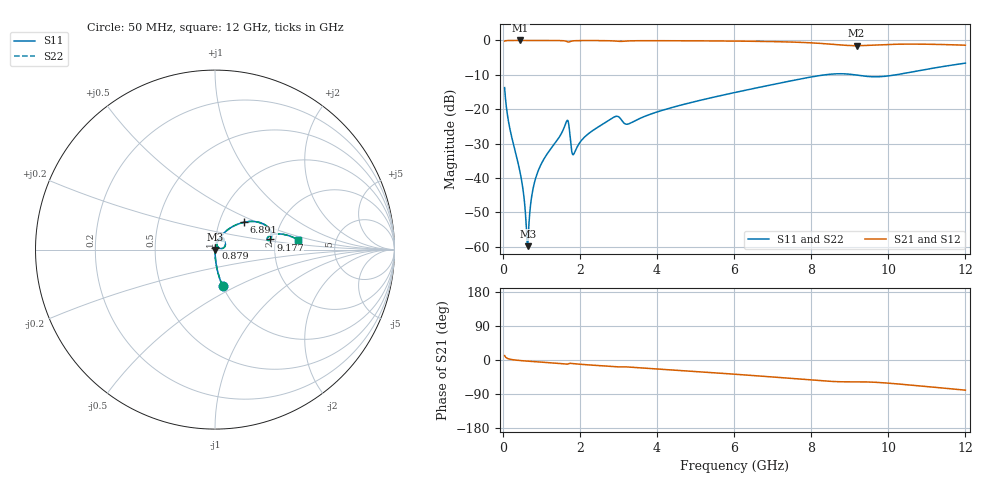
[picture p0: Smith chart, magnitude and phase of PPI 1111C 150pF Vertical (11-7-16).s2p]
# GHz S MA R 50
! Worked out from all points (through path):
!   1601 points, 50 MHz to 12 GHz, reference 50 ohm
!   highest |S21| = -0.01 dB at 453.3 MHz (marker M1); lowest = -1.5 dB at 9.177 GHz (marker M2)
!   group delay of S21, straight-line fit = 18.3 ps
!   lowest |S11| = -59.9 dB at 647.5 MHz (marker M3), VSWR 1.00, Z = 50.1 + j0.0126 ohm
!   |S11| at or under -10 dB: start of sweep to 8.361 GHz; 9.128 GHz to 10.2 GHz (1.071 GHz wide, 11.1 % of centre)
!   |S22| runs from -59.9 to -6.6 dB; largest |S21 - S12| = 0
!   S11 on the Smith chart (normalised r, x): 50 MHz: 1.00, -0.42; 879 MHz: 1.00, +0.02; 6.891 GHz: 1.31, +0.42; 9.177 GHz: 1.87, +0.24; 12 GHz: 2.70, +0.37
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0.05  0.2058 -78.3  0.9782 11.6  0.9782 11.6  0.2058 -78.3
0.1844375  0.05266 -87.2  0.998 2.2  0.998 2.2  0.05266 -87.2
0.4533125  0.01192 -87.4  0.9991 -1.4  0.9991 -1.4  0.01192 -87.4
0.5354688  0.006254 -83.7  0.999 -2.1  0.999 -2.1  0.006254 -83.7
0.6101562  0.002056 -64.5  0.999 -2.7  0.999 -2.7  0.002056 -64.5
0.6475  0.001017 7.1  0.999 -3.0  0.999 -3.0  0.001017 7.1
0.6848437  0.002311 60.2  0.9989 -3.3  0.9989 -3.3  0.002311 60.2
0.7744688  0.00639 76.1  0.9988 -4.0  0.9988 -4.0  0.00639 76.1
0.8790313  0.01092 79.0  0.9987 -4.7  0.9987 -4.7  0.01092 79.0
1.648313  0.06486 55.0  0.9719 -11.1  0.9719 -11.1  0.06486 55.0
1.700594  0.06565 27.9  0.9475 -10.3  0.9475 -10.3  0.06565 27.9
1.835031  0.02189 44.6  0.9869 -9.6  0.9869 -9.6  0.02189 44.6
2.044156  0.03521 71.3  0.9949 -11.5  0.9949 -11.5  0.03521 71.3
2.903062  0.07747 60.1  0.9808 -17.8  0.9808 -17.8  0.07747 60.1
3.239156  0.06057 55.8  0.9816 -18.4  0.9816 -18.4  0.06057 55.8
4.038312  0.09242 63.3  0.991 -23.9  0.991 -23.9  0.09242 63.3
6.025  0.175 50.5  0.9782 -37.5  0.9782 -37.5  0.175 50.5
6.891375  0.2215 43.3  0.9645 -44.0  0.9645 -44.0  0.2215 43.3
8.019156  0.2953 30.3  0.9214 -53.0  0.9214 -53.0  0.2953 30.3
9.176813  0.3136 10.4  0.8391 -57.6  0.8391 -57.6  0.3136 10.4
10.01331  0.3052 13.5  0.8746 -61.2  0.8746 -61.2  0.3052 13.5
12  0.4678 6.6  0.8524 -79.6  0.8524 -79.6  0.4678 6.6
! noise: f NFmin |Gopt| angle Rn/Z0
0.05  0.000404  0.876  0.3398  0.0007035
1.372  0.005554  0.7673  6.339  0.004842
2.701  0.01257  0.7958  12.46  0.01257
4.031  0.01308  0.7225  18.33  0.00912
5.36  0.01545  0.6971  24  0.009546
6.682  0.02336  0.7478  29.78  0.01743
8.012  0.05033  0.8544  35.71  0.06693
9.341  0.1043  0.9174  41.31  0.2441
10.67  0.07205  0.8706  46.43  0.1013
12  0.05925  0.8321  51.18  0.06066
